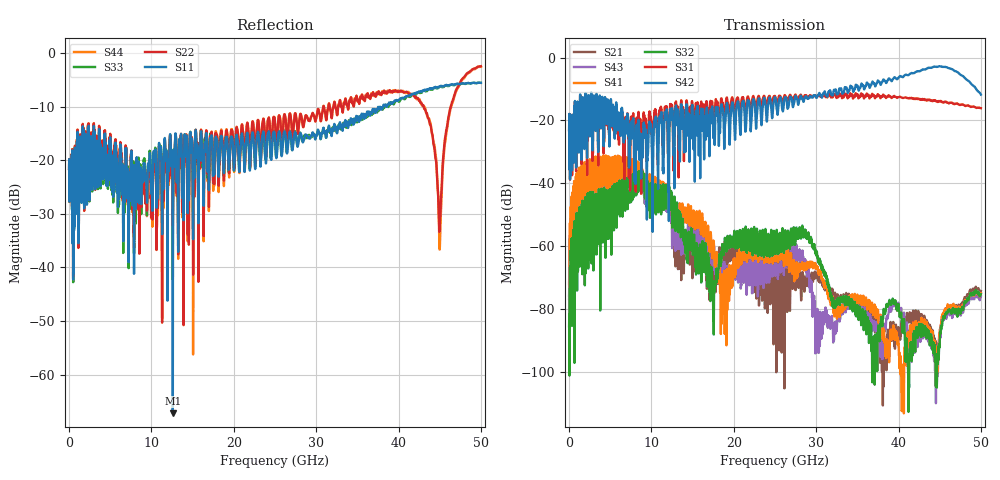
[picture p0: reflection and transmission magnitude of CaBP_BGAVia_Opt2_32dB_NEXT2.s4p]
!* Samtec Inc. NovaRay Examax Flyover System  *
!*  REV DATE  = 08/08/18  *
!*  TYPE  = TOUCHSTONE  *
!*  PORTS  = 4 port  *
!*  UNITS  = GHz  *
!*  DATA RANGE = DC  to 50 GHz; 10 MHz Step  *
!*  PARAMETER  = S  *
!*  FORMAT  = Real-Imaginary  *
!*  REFERENCE  = 50 ohms  *
!*  SOURCE  = HFSS  *
!*  VALIDATED  = No  *
!*  MANUFACTURER = SAMTEC  *
!*  INTERCONNECT = NVAx to EBCx to EBCx to NVAx  *
!*  [Full Channel NVAx to EBCx to EBCx to NVAx  with PCB Trace and BGA Via]  *
!*  BOUNDARY A  = Silicon BGA Ball Pad  *
!*  BOUNDARY B  = Silicon BGA Ball Pad  *
!*  NVAx (end a) ->>- (end b) NVAx  *
!*  Port 01 ->>- Port 02  *
!*  Port 03 ->>- Port 04  *
!***************************** CHANNEL MODEL ******************************************
# GHz S RI R 50
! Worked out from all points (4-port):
!   5000 points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, 10 MHz to 50 GHz, reference 50 ohm
!   strongest paths, dB at 10 MHz, 12.51 GHz, 25.01 GHz, 37.51 GHz, 50 GHz:
!     S42: -23.1, -16.2, -12.6, -7.3, -11.8
!     S31: -23.1, -15.2, -12.2, -11.7, -16.1
!     S32: -85.5, -47.2, -62.4, -88.8, -75.3
!     S41: -72.1, -51.2, -63.7, -80.6, -75.0
!     S43: -75.7, -55.4, -69.4, -91.5, -76.0
!     S21: -76.8, -55.6, -71.8, -84.1, -74.3
!   lowest |S11| = -67.2 dB at 12.6 GHz (marker M1), VSWR 1.00, Z = 50 + j0.0147 ohm
!   |S11| at or under -10 dB: start of sweep to 37.74 GHz; 37.74 GHz to 38.13 GHz (385.5 MHz wide, 1.02 % of centre); 38.51568 GHz to 38.54961 GHz (33.93 MHz wide, 0.0881 % of centre)
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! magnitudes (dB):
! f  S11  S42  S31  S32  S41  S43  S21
! 10 MHz  -21.6  -23.1  -23.1  -85.5  -72.1  -75.7  -76.8
! 2.7 GHz  -15.9  -11.1  -11.6  -57.4  -36.5  -41.7  -43.3
! 12.6 GHz  -67.2  -19.9  -21.8  -48.1  -49.9  -56.1  -58.0
! 18.57 GHz  -16.4  -16.2  -14.1  -61.6  -69.7  -67.0  -63.5
! 40.52 GHz  -8.4  -6.2  -12.9  -87.6  -100.8  -85.5  -85.9
! 45.02 GHz  -6.3  -2.7  -13.9  -88.3  -86.9  -88.1  -87.3
! 50 GHz  -5.5  -11.8  -16.1  -75.3  -75.0  -76.0  -74.3
